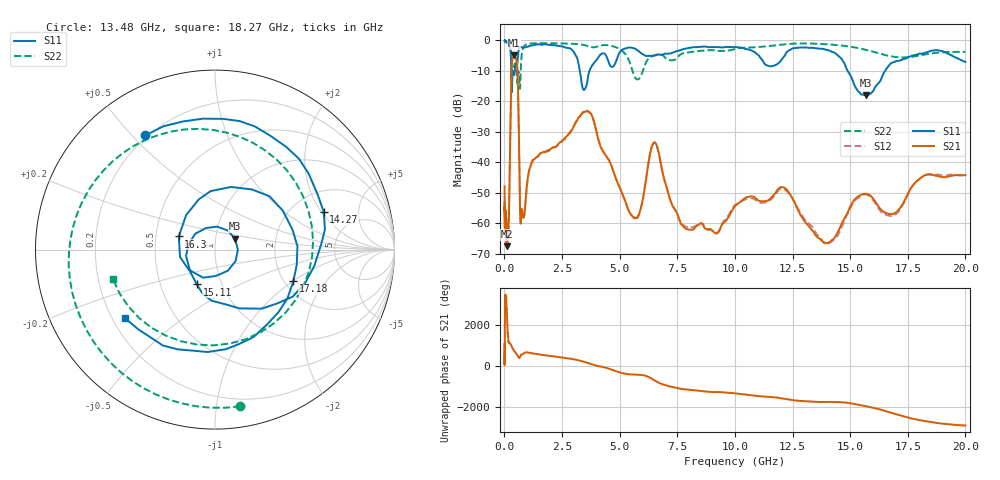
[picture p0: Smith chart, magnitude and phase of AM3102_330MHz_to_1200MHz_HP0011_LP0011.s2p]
! Date/Time: Tue, Sep 11, 2018 5:11 PM
! Network Analyzer: Agilent Technologies E8362B Rev: A.07.50.63
! Sweep from 0.010 to 20.000 GHz, 1601 Points, Sweep Type: LOG
! Power Supply: 4.950 V, 0.001 A
# Hz S DB R 50
!freq MagS11 AngS11 MagS21 AngS21 MagS12 AngS12 MagS22 AngS22
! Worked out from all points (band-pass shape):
!   1601 points, 10 MHz to 20 GHz, reference 50 ohm
!   highest |S21| = -4.88 dB at 412.5 MHz (marker M1); lowest = -67.5 dB at 111.7 MHz (marker M2)
!   |S21| within 3 dB of the highest: 323.7 MHz to 549.5 MHz (225.8 MHz wide, 51.7 % of centre)
!   lowest |S11| = -18.0 dB at 15.7 GHz (marker M3), VSWR 1.29, Z = 62 + j7.63 ohm
!   |S11| at or under -10 dB: 298.7 MHz to 439.9 MHz (141.3 MHz wide, 38.3 % of centre); 3.278 GHz to 3.69 GHz (411.3 MHz wide, 11.8 % of centre); 14.89 GHz to 16.51 GHz (1.621 GHz wide, 10.3 % of centre)
!   |S22| runs from -15.9 to -0.2 dB; largest |S21 - S12| = 0.0089
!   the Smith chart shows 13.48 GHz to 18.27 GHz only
!   S11 on the Smith chart (normalised r, x): 13.48 GHz: 0.19, +0.54; 14.27 GHz: 2.96, +2.10; 15.11 GHz: 0.76, -0.31; 16.3 GHz: 0.66, +0.10; 17.18 GHz: 2.24, -1.01; 18.27 GHz: 0.25, -0.32
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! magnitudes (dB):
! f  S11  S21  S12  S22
! 10 MHz  0.0  -47.9  -53.7  -0.2
! 35.55 MHz  0.0  -59.4  -61.3  -0.4
! 111.7 MHz  -0.4  -67.5  -63.2  -0.8
! 126.4 MHz  -0.4  -63.4  -64.1  -0.9
! 185.7 MHz  -1.0  -60.0  -62.6  -1.2
! 412.5 MHz  -11.3  -4.9  -4.9  -8.7
! 447.2 MHz  -9.6  -5.1  -5.2  -7.7
! 572.5 MHz  -6.8  -11.0  -11.2  -13.4
! 702.3 MHz  -2.2  -59.7  -59.9  -11.7
! 1.59 GHz  -1.4  -36.9  -37.0  -0.9
! 3.651 GHz  -11.0  -23.4  -23.2  -1.9
! 5.652 GHz  -2.7  -58.2  -58.6  -11.9
! 6.518 GHz  -4.9  -33.4  -33.6  -4.9
! 7.92 GHz  -2.6  -61.9  -61.1  -4.0
! 13.48 GHz  -2.5  -63.7  -62.7  -1.1
! 14.27 GHz  -3.9  -65.2  -65.6  -1.4
! 15.11 GHz  -13.2  -53.1  -53.4  -2.2
! 15.7 GHz  -18.0  -50.3  -50.6  -3.1
! 16.3 GHz  -13.4  -55.2  -55.9  -4.3
! 17.18 GHz  -6.5  -54.9  -55.4  -5.6
! 18.27 GHz  -4.0  -44.1  -44.1  -4.6
! 20 GHz  -7.1  -44.2  -44.4  -3.7
